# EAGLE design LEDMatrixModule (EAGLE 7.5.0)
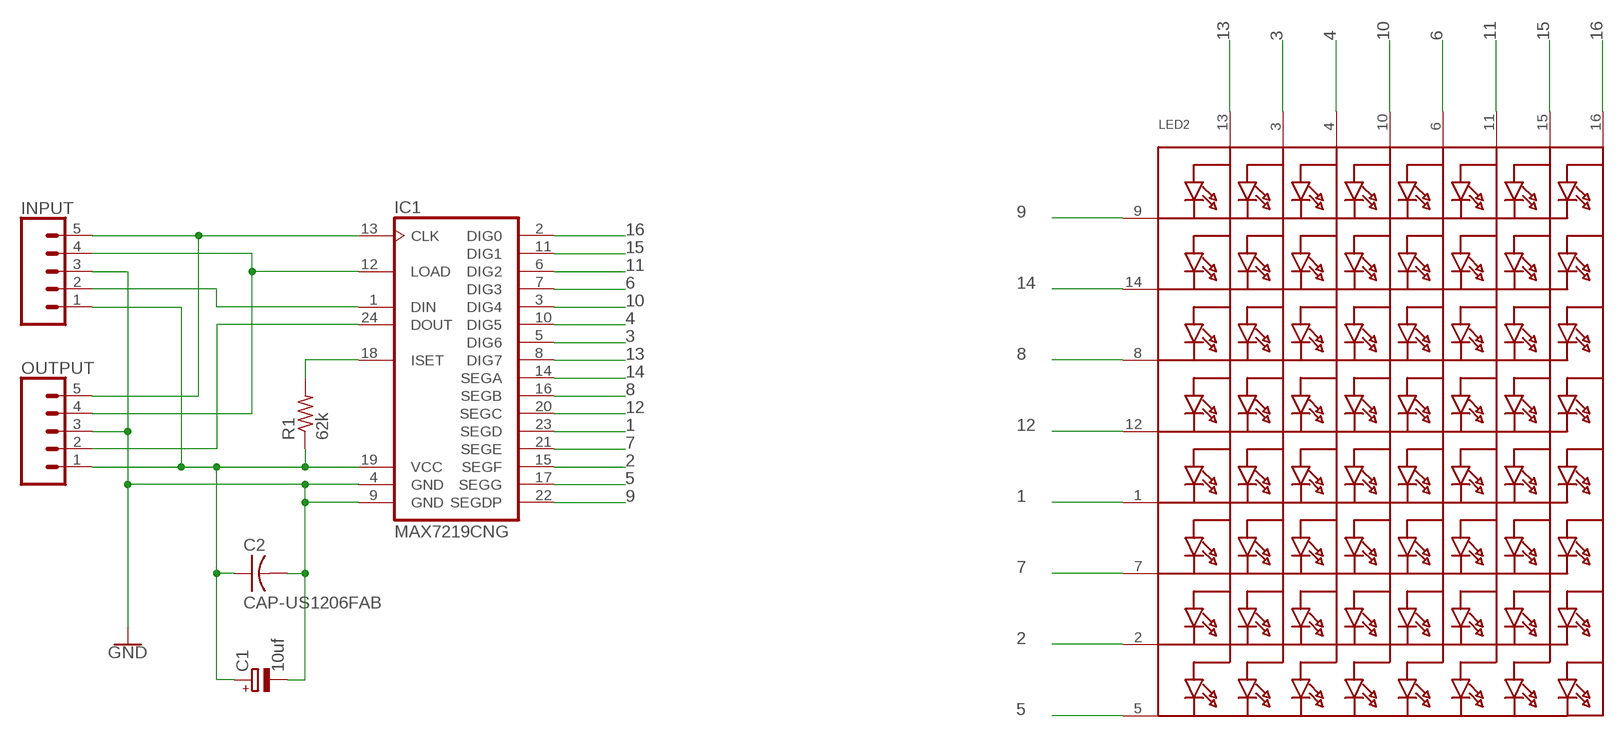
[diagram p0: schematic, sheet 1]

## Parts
C1  10uf  CPOL-EUE2.5-6  [E2,5-6]
C2  CAP-US1206FAB  [C1206FAB]
IC1  MAX7219CNG  [DIL24-3]
INPUT  CONN_05  [1X05]
LED2  SEGMENT_8X8_ROWCATHODEBL-M15  [SEGMENT_BL-M15A881]
OUTPUT  CONN_05  [1X05]
R1  62k  R-US_0309/10  [0309/10]

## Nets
1: IC1.23(SEGD) LED2.1(K5)
2: IC1.15(SEGF) LED2.2(K7)
3: IC1.5(DIG6) LED2.3(A2)
4: IC1.10(DIG5) LED2.4(A3)
5: IC1.17(SEGG) LED2.5(K8)
6: IC1.7(DIG3) LED2.6(A5)
7: IC1.21(SEGE) LED2.7(K6)
8: IC1.16(SEGB) LED2.8(K3)
9: IC1.22(SEGDP) LED2.9(K1)
10: IC1.3(DIG4) LED2.10(A4)
11: IC1.6(DIG2) LED2.11(A6)
12: IC1.20(SEGC) LED2.12(K4)
13: IC1.8(DIG7) LED2.13(A1)
14: IC1.14(SEGA) LED2.14(K2)
15: IC1.11(DIG1) LED2.15(A7)
16: IC1.2(DIG0) LED2.16(A8)
GND: C1.- C2.2 IC1.4(GND) IC1.9(GND) INPUT.3 OUTPUT.3
N$1: IC1.13(CLK) INPUT.5 OUTPUT.5
N$2: C1.+ C2.1 IC1.19(VCC) INPUT.1 OUTPUT.1 R1.1
N$3: IC1.18(ISET) R1.2
N$4: IC1.24(DOUT) OUTPUT.2
N$5: IC1.1(DIN) INPUT.2
N$6: IC1.12(LOAD) INPUT.4 OUTPUT.4

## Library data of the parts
C1 = rcl:CPOL-EU: POLARIZED CAPACITOR, European symbol
C2 = fab:CAP-US
IC1 = max7219:MAX7219CNG: LED DISPLAY DRIVER; MF: MAXIM; MPN: MAX7219CNG; OC_FARNELL: 1523914; OC_NEWARK: 34C4018
INPUT OUTPUT = SparkFun-Connectors:CONN_05: Multi connection point. Often used as Generic Header-pin footprint for 0.1 inch spaced/style header connections On any of the 0.1 inch spaced packages, you can populate with these: Break Away Headers - Straight (PRT-00116) Break Away Male Headers - Right Angle (PRT-00553) Female Headers (PRT-00115)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
LED2 = adafruit:SEGMENT_8X8_ROWCATHODE: 8x8 LED Segment Displays: Row = Cathode 0.7" Red 8X8 Matrix, 1.9mm Round LEDs - BL-M07C881UR 1.2" Red 8x8 Matrix, 3.0mm Round LEDs - BL-M12A881UR 1.2" Red 8x8 Matrix, 3.0mm Square LEDs - BL-M12A883
R1 = BeagleBone_Black_Wireless:R-US_: RESISTOR, American symbol

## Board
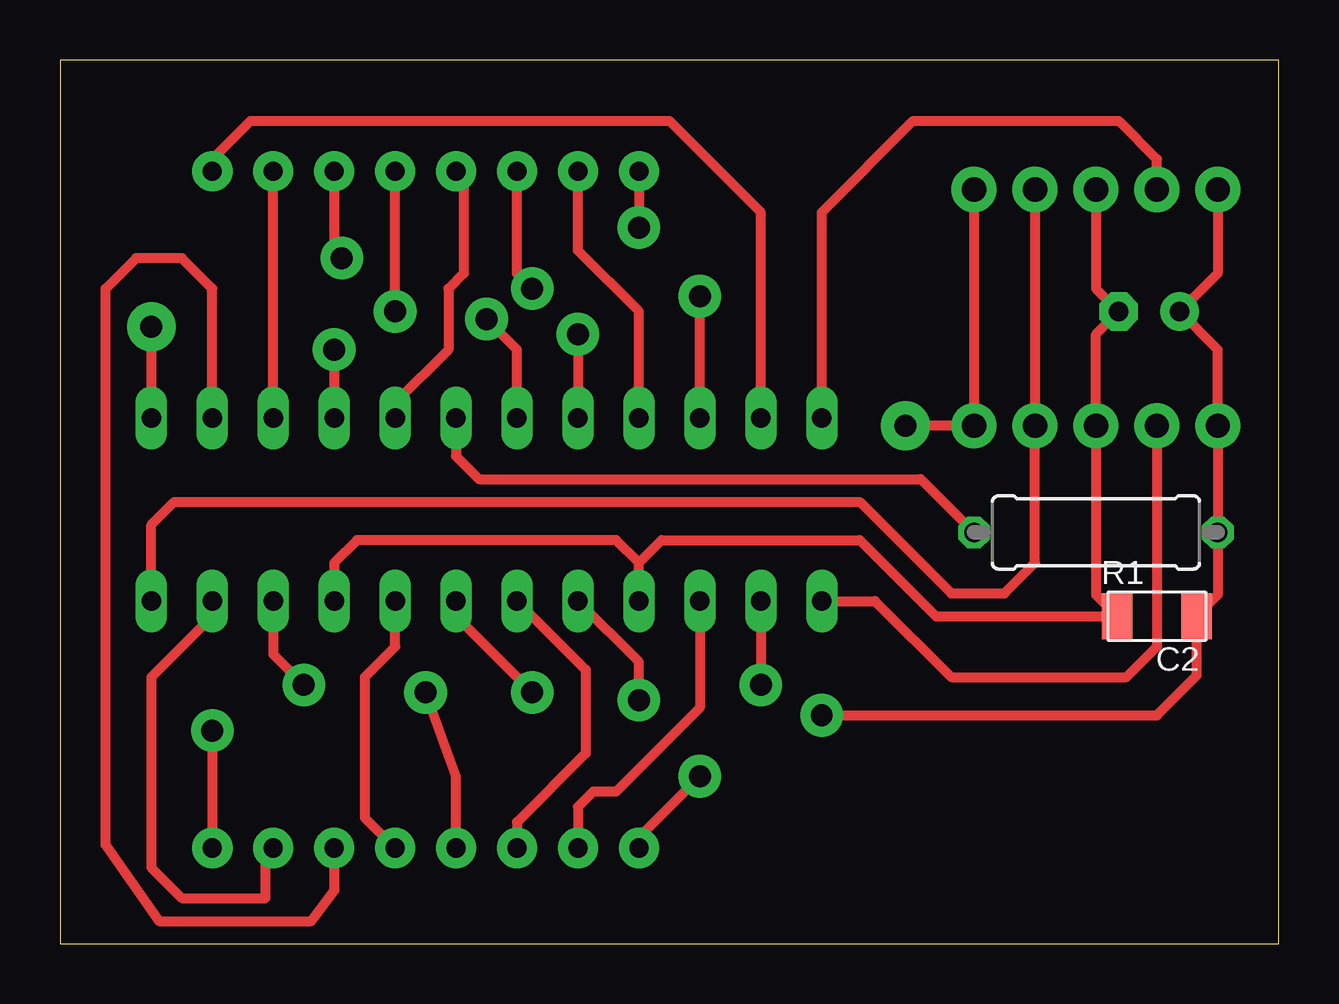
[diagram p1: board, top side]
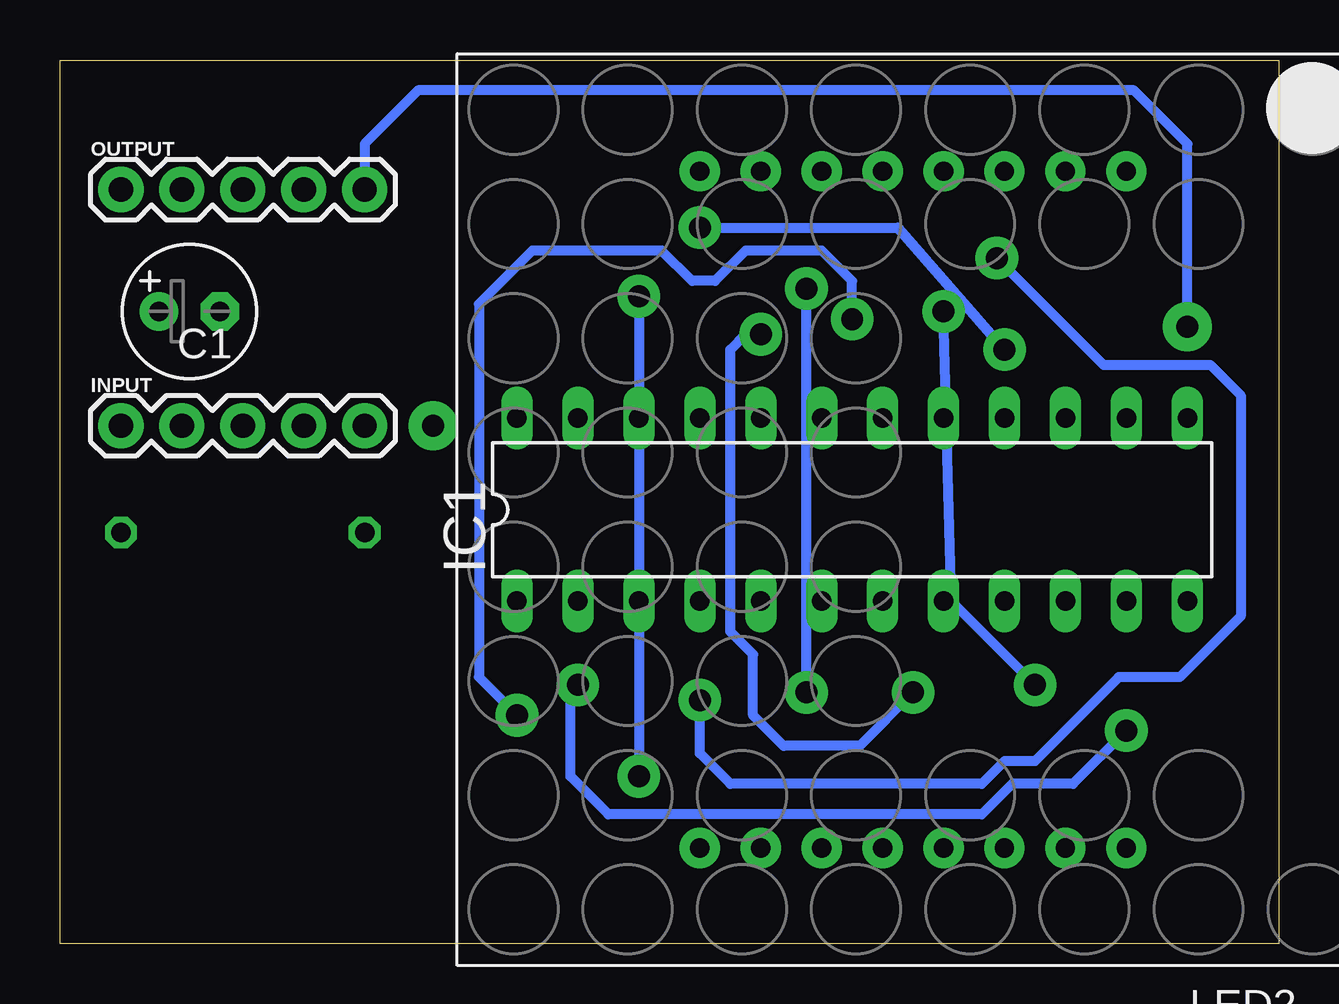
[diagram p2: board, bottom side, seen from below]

Size 50.8 x 36.83 mm. Coordinates in mm from the lower left corner, seen from the top.
Outline: 0,0 50.8,0 50.8,36.83 0,36.83 0,0
Copper layers (1*16): Top 0.035mm / dielectric 1.5mm / Bottom 0.035mm
Design rules "default": minimum track width 10mil, minimum drill 24mil, track to track 8mil, track to pad 8mil, pad to pad 8mil, via to via 8mil, smd to smd 8mil, copper to edge 40mil, drill to drill 8mil, minimum pad ring 10mil, minimum via ring 8mil, stop-mask expansion 4mil, vias tented up to drill 0mil, thermal gap 10mil

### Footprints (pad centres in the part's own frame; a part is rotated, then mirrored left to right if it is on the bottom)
E2,5-6 = drill 0.813 pad 1.6: + -1.27,0 | drill 0.813 pad 1.6 octagon: - 1.27,0
C1206FAB = smd 1.27 x 1.905: 1 -1.651,0; 2 1.651,0
DIL24-3 = drill 0.813 long: 1 -13.97,-3.81; 2 -11.43,-3.81; 3 -8.89,-3.81; 4 -6.35,-3.81; 5 -3.81,-3.81; 6 -1.27,-3.81; 7 1.27,-3.81; 8 3.81,-3.81; 9 6.35,-3.81; 10 8.89,-3.81; 11 11.43,-3.81; 12 13.97,-3.81; 13 13.97,3.81; 14 11.43,3.81; 15 8.89,3.81; 16 6.35,3.81; 17 3.81,3.81; 18 1.27,3.81; 19 -1.27,3.81; 20 -3.81,3.81; 21 -6.35,3.81; 22 -8.89,3.81; 23 -11.43,3.81; 24 -13.97,3.81
1X05 = drill 1.016 pad 1.88: 1 0,0; 2 2.54,0; 3 5.08,0; 4 7.62,0; 5 10.16,0
SEGMENT_BL-M15A881 = drill 0.8 pad 1.676: 1 -8.89,-14.1; 2 -6.35,-14.1; 3 -3.81,-14.1; 4 -1.27,-14.1; 5 1.27,-14.1; 6 3.81,-14.1; 7 6.35,-14.1; 8 8.89,-14.1; 9 8.89,14.1; 10 6.35,14.1; 11 3.81,14.1; 12 1.27,14.1; 13 -1.27,14.1; 14 -3.81,14.1; 15 -6.35,14.1; 16 -8.89,14.1
0309/10 = drill 0.813 octagon: 1 -5.08,0; 2 5.08,0

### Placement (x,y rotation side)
C1  45.4,26.35 0 bottom
C2  45.72,13.65 180 top
IC1  17.78,18.1 0 bottom
INPUT  48.26,21.59 0 bottom
LED2  15.24,18.1 180 bottom
OUTPUT  48.26,31.43 0 bottom
R1  43.18,17.14 180 top

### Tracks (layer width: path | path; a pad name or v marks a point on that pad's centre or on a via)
1
  Top 0.406: IC1.23 29.21,30.48 25.4,34.29 7.94,34.29 6.35,32.7 LED2.1
2
  Top 0.406: IC1.15 LED2.2
3  (via drill 0.91 pad 1.78)
  Top 0.406: LED2.3 11.43,28.89 v11.75,28.57 | v24.13,10.16 24.13,11.75 IC1.5
  Bottom 0.406: v11.75,28.57 7.3,24.13 2.86,24.13 1.59,22.86 1.59,13.65 4.13,11.11 6.67,11.11 10.16,7.62 11.43,7.62 12.38,6.67 22.86,6.67 24.13,7.94 v24.13,10.16
4  (via drill 0.91 pad 1.78)
  Top 0.406: IC1.10 8.89,12.06 v10.16,10.79 | v13.97,26.35 LED2.4
  Bottom 0.406: v10.16,10.79 13.65,14.29 v13.97,26.35
5
  Top 0.406: LED2.5 16.83,31.88 16.83,27.94 16.19,27.3 16.19,24.77 13.97,22.54 IC1.17
6  (via drill 0.91 pad 1.78)
  Top 0.406: IC1.7 16.51,13.65 v19.68,10.48 | v19.68,27.3 19.05,27.94 LED2.6
  Bottom 0.406: v19.68,10.48 v19.68,27.3
7
  Top 0.406: IC1.21 24.13,26.35 21.59,28.89 LED2.7
8  (via drill 0.91 pad 1.78)
  Top 0.406: LED2.8 v24.13,29.84 | v11.43,24.77 IC1.16
  Bottom 0.406: v24.13,29.84 15.88,29.84 v11.43,24.77
9  (via drill 0.91 pad 1.78)
  Top 0.406: IC1.22 v26.67,26.99 | LED2.9 24.13,4.45 v26.67,6.99
  Bottom 0.406: v26.67,26.99 v26.67,6.99
10
  Top 0.406: IC1.3 26.67,9.84 23.18,6.35 22.23,6.35 21.59,5.71 LED2.10
11
  Top 0.406: IC1.6 21.91,11.43 21.91,7.94 19.05,5.08 LED2.11
12  (via drill 0.91 pad 1.78)
  Top 0.406: v21.59,25.4 IC1.20 | LED2.12 16.51,6.99 v15.24,10.48
  Bottom 0.406: v15.24,10.48 17.46,8.26 20.64,8.26 21.91,9.53 21.91,12.06 22.86,13.02 22.86,24.77 22.23,25.4 v21.59,25.4
13
  Top 0.406: LED2.13 12.7,5.27 12.7,11.11 13.97,12.38 IC1.8
14
  Top 0.406: LED2.14 11.43,2.22 10.48,0.95 4.13,0.95 1.91,4.13 1.91,27.3 3.17,28.57 5.08,28.57 6.35,27.3 IC1.14
15
  Top 0.406: IC1.11 6.35,13.65 3.81,11.11 3.81,3.17 5.08,1.91 8.57,1.91 8.57,3.68 LED2.15
16  (via drill 0.91 pad 1.78)
  Top 0.406: IC1.2 v29.21,10.79 | v6.35,8.89 LED2.16
  Bottom 0.406: v29.21,10.79 29.21,10.16 29.53,10.16 29.53,6.99 27.94,5.4 12.38,5.4 11.11,6.67 8.57,6.67 v6.35,8.89
GND
  Top 0.406: OUTPUT.3 43.18,27.3 C1.- 43.18,25.4 INPUT.3 43.18,14.54 C2.2 | C2.2 44.07,13.27 | 24.13,15.88 25.08,16.83 33.34,16.83 36.51,13.65 C2.2 | IC1.4 24.13,15.88 | 24.13,15.88 23.18,16.83 12.38,16.83 11.43,15.88 IC1.9
N$1  (via drill 0.91 pad 2.03)
  Top 0.406: OUTPUT.5 INPUT.5 v35.24,21.59 | v3.81,25.72 IC1.13
  Bottom 0.406: v3.81,25.72 3.81,33.34 6.03,35.56 35.88,35.56 38.1,33.34 OUTPUT.5
N$2  (via drill 0.91 pad 1.78)
  Top 0.406: OUTPUT.1 48.26,27.94 C1.+ 48.26,24.77 INPUT.1 R1.1 48.26,14.54 C2.1 47.37,11.18 45.72,9.53 v31.75,9.53 | IC1.19 19.05,24.77 v17.78,26.04
  Bottom 0.406: v17.78,26.04 17.78,27.62 19.05,28.89 22.23,28.89 23.5,27.62 24.45,27.62 25.72,28.89 31.11,28.89 33.34,26.67 33.34,11.11 v31.75,9.53
N$3
  Top 0.406: IC1.18 16.51,20.32 17.46,19.37 35.88,19.37 R1.2
N$4
  Top 0.406: OUTPUT.2 45.72,32.7 44.13,34.29 35.56,34.29 31.75,30.48 IC1.24
N$5
  Top 0.406: INPUT.2 45.72,12.38 44.45,11.11 37.15,11.11 33.97,14.29 IC1.1
N$6
  Top 0.406: OUTPUT.4 INPUT.4 40.64,15.88 39.37,14.61 37.15,14.61 33.34,18.41 4.76,18.41 3.81,17.46 IC1.12

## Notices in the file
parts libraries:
SparkFun-Connectors: Licensing: Creative Commons ShareAlike 4.0 International - https://creativecommons.org/licenses/by-sa/4.0
